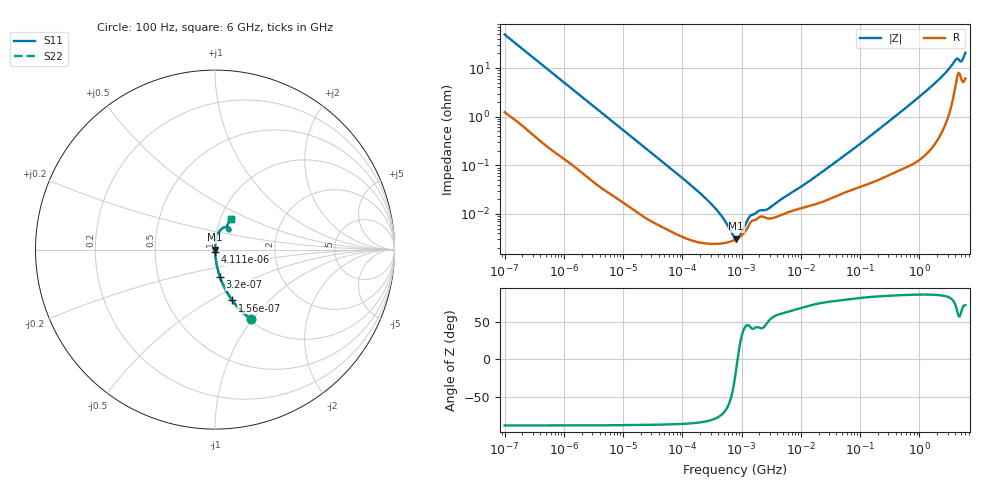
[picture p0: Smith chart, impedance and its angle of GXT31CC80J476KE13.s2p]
!Murata Part Number: GXT31CC80J476KE13
!These Parameters are Measured in Series Mode Connection
!Data Generated on Jan 08, 2026
!  o--ll--o
!Port1  Port2
!  o------o
!Operation Temp=25[degC], DC Bias Voltage=0[V]
!Freq. Start=100[Hz] Stop=6[GHz] 401[Steps]
# Hz S RI R 50
!Freq.(Hz) S11(Real) S11(Imag) S21(Real) S21(Imag) S12(Real) S12(Imag) S22(Real) S22(Imag)
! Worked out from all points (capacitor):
!   401 points, 100 Hz to 6 GHz, reference 50 ohm
!   read as one part in series: C = 32.2 uF near 109 Hz
!   lowest |Z| = 3.1 mohm at 810.1 kHz (marker M1)
!   series resonance near 854.2 kHz, so ESL is about 1.1 nH
!   S11 on the Smith chart (normalised r, x): 100 Hz: 1.02, -0.98; 156 Hz: 1.02, -0.63; 320 Hz: 1.01, -0.31; 4.111 kHz: 1.00, -0.03; 6 GHz: 1.12, +0.40
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100  0.2005 -0.3879  0.7995 0.3879  0.7995 0.3879  0.2005 -0.3879
156  0.0971 -0.2833  0.9029 0.2833  0.9029 0.2833  0.0971 -0.2833
320  0.0276 -0.1516  0.9724 0.1516  0.9724 0.1516  0.0276 -0.1516
717  0.00676 -0.0701  0.9932 0.0701  0.9932 0.0701  0.00676 -0.0701
2008  0.00137 -0.0257  0.9986 0.0257  0.9986 0.0257  0.00137 -0.0257
4111  0.000516 -0.0127  0.9995 0.0127  0.9995 0.0127  0.000516 -0.0127
40335  5.97e-05 -0.00135  0.9999 0.00135  0.9999 0.00135  5.97e-05 -0.00135
184852  2.63e-05 -0.000289  1 0.000289  1 0.000289  2.63e-05 -0.000289
432798  2.45e-05 -9.68e-05  1 9.68e-05  1 9.68e-05  2.45e-05 -9.68e-05
774597  2.94e-05 -1.31e-05  1 1.31e-05  1 1.31e-05  2.94e-05 -1.31e-05
810067  3.02e-05 -7.1e-06  1 7.1e-06  1 7.1e-06  3.02e-05 -7.1e-06
1585629  7.37e-05 6.44e-05  0.9999 -6.44e-05  0.9999 -6.44e-05  7.37e-05 6.44e-05
2074311  8.8e-05 7.96e-05  0.9999 -7.96e-05  0.9999 -7.96e-05  8.8e-05 7.96e-05
2713602  8.15e-05 9.46e-05  0.9999 -9.46e-05  0.9999 -9.46e-05  8.15e-05 9.46e-05
1.555665e7  0.000151 0.000499  0.9998 -0.000499  0.9998 -0.000499  0.000151 0.000499
7.797396e7  0.000327 0.00217  0.9997 -0.00217  0.9997 -0.00217  0.000327 0.00217
3.124326e8  0.000699 0.00814  0.9993 -0.00814  0.9993 -0.00814  0.000699 0.00814
1.791126e9  0.00487 0.0471  0.9951 -0.0471  0.9951 -0.0471  0.00487 0.0471
2.679998e9  0.012 0.0749  0.988 -0.0749  0.988 -0.0749  0.012 0.0749
4.009986e9  0.0535 0.1252  0.9465 -0.1252  0.9465 -0.1252  0.0535 0.1252
5.016141e9  0.072 0.1041  0.928 -0.1041  0.928 -0.1041  0.072 0.1041
6e9  0.0895 0.1704  0.9105 -0.1704  0.9105 -0.1704  0.0895 0.1704
